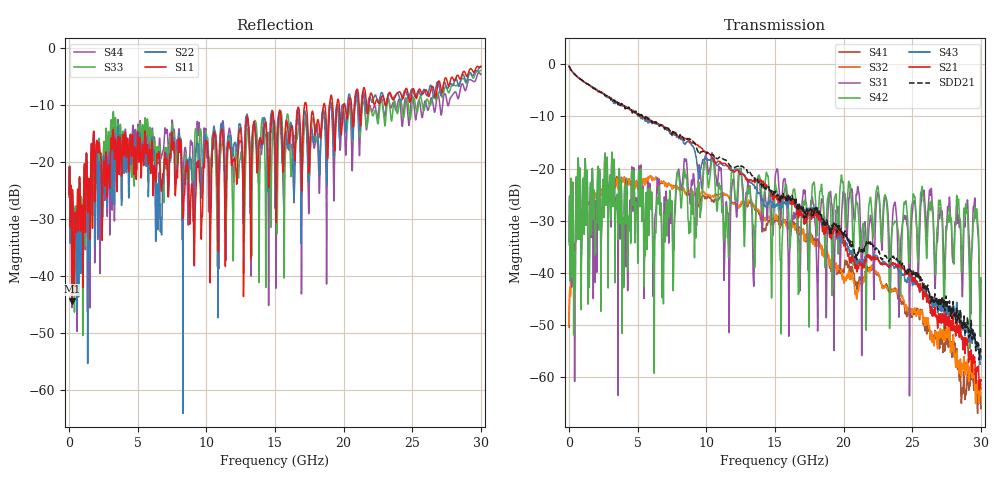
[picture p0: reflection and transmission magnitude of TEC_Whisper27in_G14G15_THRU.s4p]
! Tyco Electronics
! G14G15_THRU
!! PART DESCRIPTION: Whisper 27in Megtron 6 VLP-HVLP-VLP Channel Model, bulkhead 2.4mm test pts
!! MODEL DESCRIPTION: System 4-port S-parameter
!! MODEL STATUS: Measured
!! MODEL GEOMETRY: Channel Model
!! MODEL FREQUENCY RANGE: DC to 30.000 GHz in 10.000 MHz frequency steps
!! MODEL EDGE RATE LIMITATION: 12.500 ps (Using conservative 0.5/Fmax rule of thumb)
!! TIME-DOMAIN TRANSFORM CAUTIONS:
!! 1.) Do not simulate transient edge rates faster than the number listed above.  Edge rates faster than this number
!!  contain significant spectral content at frequencies above the model's highest frequency.
!! 2.) Even when simulating edge rates that are slower than the number listed above, be aware that the best time
!!  resolution possible with a direct iFFT is (1 / 2Fmax).  As a result, time resolution is typically not adequate
!!  for most time-domain simulations unless tricks such as windowing are used to minimize leakage and aliasing.
!! 3.) Because the model has a uniform frequency step, a direct iFFT will result in an impulse that that has a time
!!  length given by either (1 / Fstep) or (1 / 2Fstep), depending on the transform being used.  Care has been taken
!!  in selecting the frequency step to ensure a settled impulse response for the model.  Therefore, convolution with
!!  the model's impulse response should present no issues.  However, if directly concatenating s-parameter models
!!  in the frequency domain a user must either interpolate necessary interim frequencies or complete impulse response
!!  zero-padding.  Impulse response zero-padding is more difficult, but more accurate.
!! PORT DEFINITIONS:
!! Port  1  ----->  Side A  G14  Side B  <-----  Port  2
!! Port  3  ----->  Side A  G15  Side B  <-----  Port  4
! Point-to-Point link (differential)  !
! Connectors:  !
!  1: STRADA Whisper  !
! Materials:  !
!  Backplane: Megtron-6 HVLP  !
!  Daughtercard: Megtron-6 VLP  !
! Stack-up:  !
!  Backplane: 20 layers, 200mil thick  !
!  Daughtercard: 14 layers, 110mil thick  !
! Trace Length:  !
!  Backplane: 17in  !
!  Daightercards: 5in  !
! Trace Width:  !
!  Backplane: 8-13-8 mils  !
!  Daughtercards: 6-9-6 mils  !
! Geometry:  !
!  Backplane: Stripline  !
!  Daughtercards: Stripline  !
! Layer Connections:  !
!  Backplane: Layer 16, counterbored(1-6mil stub)  !
!  Daughtercard: Layer 9, counterbored(1-6mil stub) !
! Freq. Range: 0 GHz - 30 GHz  !
! Note1: non-mixed-mode s-parameters  !
! Note2: channel includes 2.4mm test points  !
! Touchstone data converted from IdEM dataset
# GHz S MA R 50
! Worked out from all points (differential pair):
!   3000 points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, 10 MHz to 30 GHz, reference 50 ohm
!   strongest paths, dB at 10 MHz, 7.51 GHz, 15.01 GHz, 22.51 GHz, 30 GHz:
!     S21: -0.4, -13.4, -25.3, -37.3, -60.5
!     S43: -0.4, -13.7, -27.2, -37.1, -56.5
!     S42: -34.6, -27.6, -22.8, -23.6, -41.0
!     S31: -33.9, -28.3, -22.1, -24.5, -41.4
!     S32: -49.8, -23.9, -29.5, -40.0, -62.0
!     S41: -50.4, -23.8, -29.9, -40.2, -66.0
!   taken as a pair (ports 1,3 in; 2,4 out), SDD21 dB: -0.3, -13.4, -24.6, -35.4, -55.2
!   lowest |S11| = -44.4 dB at 200 MHz (marker M1), VSWR 1.01, Z = 50.2 - j0.56 ohm
!   |S11| at or under -10 dB: start of sweep to 17.15 GHz; 17.28 GHz to 18.55 GHz (1.266 GHz wide, 7.06 % of centre); 18.63 GHz to 18.99 GHz (358 MHz wide, 1.9 % of centre)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
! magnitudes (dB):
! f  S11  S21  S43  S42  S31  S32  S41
! 10 MHz  -25.7  -0.4  -0.4  -34.6  -33.9  -49.8  -50.4
! 200 MHz  -44.4  -1.3  -1.3  -32.6  -32.7  -39.2  -39.0
! 3.28 GHz  -17.7  -7.0  -7.3  -18.2  -18.7  -22.7  -22.1
! 13.22 GHz  -31.4  -22.2  -22.7  -25.5  -25.1  -26.0  -26.3
! 18.1 GHz  -12.7  -28.5  -28.0  -31.5  -47.5  -34.0  -33.6
! 29.57 GHz  -4.0  -57.3  -51.7  -27.4  -25.9  -60.5  -59.5
! 30 GHz  -3.2  -60.5  -56.5  -41.0  -41.4  -62.0  -66.0
